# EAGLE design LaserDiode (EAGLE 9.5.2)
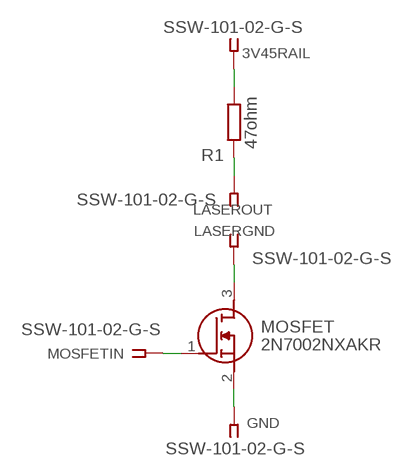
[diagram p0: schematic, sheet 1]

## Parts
3V45RAIL  SSW-101-02-G-S  [SSW-101-02-G-S]
GND  SSW-101-02-G-S  [SSW-101-02-G-S]
LASERGND  SSW-101-02-G-S  [SSW-101-02-G-S]
LASEROUT  SSW-101-02-G-S  [SSW-101-02-G-S]
MOSFET  2N7002NXAKR  [SOT95P230X110-3N]
MOSFETIN  SSW-101-02-G-S  [SSW-101-02-G-S]
R1  47ohm  R-EU_R1206  [R1206]

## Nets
N$1: MOSFET.1(G) MOSFETIN.1
N$2: GND.1 MOSFET.2(S)
N$3: 3V45RAIL.1 R1.2
N$4: LASEROUT.1 R1.1
N$5: LASERGND.1 MOSFET.3(D)

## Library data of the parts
3V45RAIL GND LASERGND LASEROUT MOSFETIN = con-samtec:SSW-101-02-G-S: THROUGH-HOLE .025" SQ POST SOCKET; MF: Samtec Inc.; MPN: SSW-101-02-G-S; OC_FARNELL: unknown; OC_NEWARK: 11P9336
MOSFET = SamacSys_Parts:2N7002NXAKR: NEXPERIA - 2N7002NXAKR - MOSFET Transistor, Trench, N Channel, 190 mA, 60 V, 3 ohm, 10 V, 1.6 V Source: Datasheet; DESCRIPTION: NEXPERIA - 2N7002NXAKR - MOSFET Transistor, Trench, N Channel, 190 mA, 60 V, 3 ohm, 10 V, 1.6 V; HEIGHT: 1.1mm; MANUFACTURER_NAME: Nexperia; MANUFACTURER_PART_NUMBER: 2N7002NXAKR; MOUSER_PART_NUMBER: 771-2N7002NXAKR; MOUSER_PRICE-STOCK: https://www.mouser.com/Search/Refine.aspx?Keyword=771-2N7002NXAKR
R1 = resistor:R-EU_: RESISTOR, European symbol

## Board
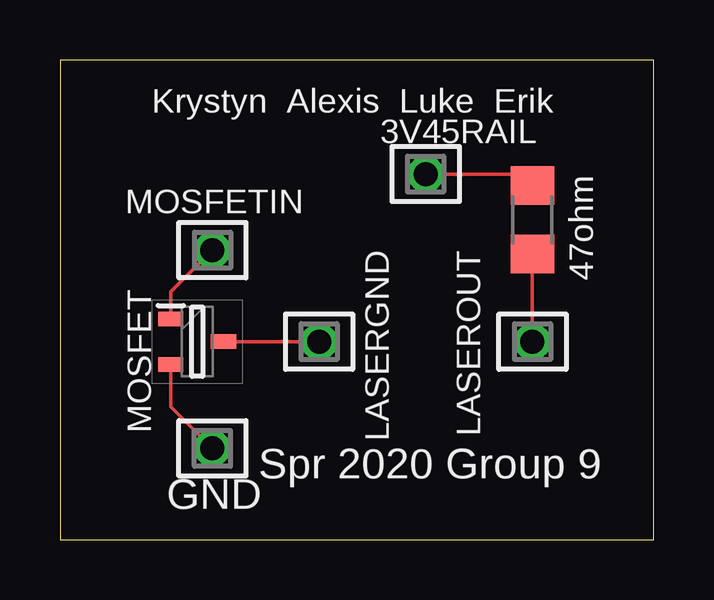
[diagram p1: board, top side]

Size 24.74 x 19.99 mm. Coordinates in mm from the lower left corner, seen from the top.
Outline: 0,0 24.74,0 24.74,19.99 0,19.99 0,0
Copper layers (1*16): Top 0.035mm / dielectric 1.5mm / Bottom 0.035mm
Design rules "default": minimum track width 6mil, minimum drill 0.35mm, track to track 6mil, track to pad 6mil, pad to pad 6mil, via to via 6mil, smd to smd 6mil, copper to edge 40mil, drill to drill 6mil, minimum pad ring 10mil, minimum via ring 8mil, stop-mask expansion 4mil, vias tented up to drill 0mil, thermal gap 10mil

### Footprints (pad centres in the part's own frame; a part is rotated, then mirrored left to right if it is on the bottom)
SSW-101-02-G-S = drill 1 pad 1.5 octagon: 1 0,0
SOT95P230X110-3N = smd 1.05 x 0.6: 1 -1.1,0.95; 2 -1.1,-0.95; 3 1.1,0
R1206 = smd 1.6 x 1.803: 1 -1.422,0; 2 1.422,0

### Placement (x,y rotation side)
3V45RAIL  15.24,15.24 180 top
GND  6.35,3.81 180 top
LASERGND  10.79,8.25 0 top
LASEROUT  19.68,8.25 0 top
MOSFET  5.71,8.25 0 top
MOSFETIN  6.35,12.07 0 top
R1  19.68,13.34 90 top

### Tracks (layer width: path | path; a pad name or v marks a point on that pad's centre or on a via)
N$1
  Top 0.152: MOSFETIN.1 4.62,10.33 MOSFET.1
N$2
  Top 0.152: MOSFET.2 4.62,5.55 GND.1
N$3
  Top 0.152: 3V45RAIL.1 19.2,15.24 R1.2
N$4
  Top 0.152: R1.1 LASEROUT.1
N$5
  Top 0.152: LASERGND.1 MOSFET.3

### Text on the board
tNames: Krystyn Alexis Luke Erik | MOSFET | Spr 2020 Group 9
